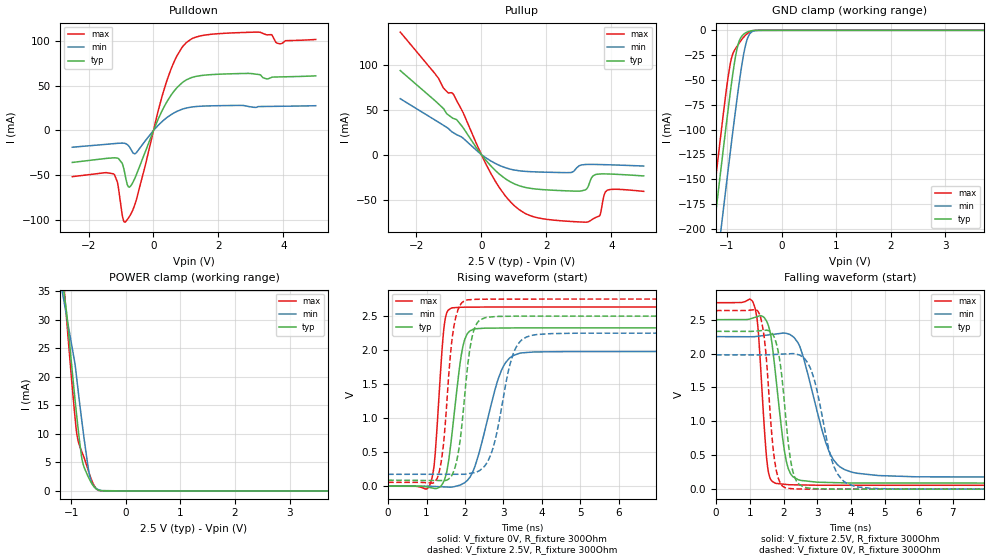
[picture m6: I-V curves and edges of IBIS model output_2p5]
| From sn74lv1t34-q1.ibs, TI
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[Model]   output_2p5
Model_type   Output
Polarity   Non-Inverting
Vmeas = 0.9
Vref = 0.9
Cref = 15pF
Rref = 100000
|   typ   min   max
C_comp   4.947pF   4.835pF   5.043pF
[Voltage Range]   2.5   2.25   2.75
[Temperature Range]   27   125   -40
[Pullup Reference]   2.5   2.25   2.75
[Pulldown Reference]   -0   0   0
[Power Clamp Reference]   2.5   2.25   2.75
[GND Clamp Reference]   0   0   0
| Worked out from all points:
|   slope of the pulldown table from 0 to 0.375 V, typ, clamps not added: 12.6 ohm
|   slope of the pullup table from 0 to 0.375 V, typ, clamps not added: 24 ohm
|   GND clamp passes 1 mA (typ) near -0.59 V on its own axis
|   POWER clamp passes 1 mA (typ) near -0.60 V on its own axis
|   falling waveform, V_fixture 2.5V, R_fixture 300Ohm: 20-80 % time 335ps typ, 676ps min, 207ps max; typ from 2.5 V to 0.088 V
|   rising waveform, V_fixture 0V, R_fixture 300Ohm: 20-80 % time 290ps typ, 552ps min, 186ps max; typ from 0 V to 2.33 V
|   rising waveform, V_fixture 2.5V, R_fixture 300Ohm: 20-80 % time 280ps typ, 452ps min, 240ps max; typ from 0.088 V to 2.5 V
|   falling waveform, V_fixture 0V, R_fixture 300Ohm: 20-80 % time 298ps typ, 523ps min, 252ps max; typ from 2.33 V to 0 V
[Pulldown]
|   Voltage   I(typ)   I(min)   I(max)
-2.5V     -35.79mA   -18.74mA   -51.7mA
-1.23V    -30.63mA   -14.75mA   -48.54mA
-1.114V   -30.88mA   -14.41mA   -57.55mA
-956.5mV  -37.5mA    -14.14mA   -95.94mA
-872.5mV  -50.05mA   -14.51mA   -102.7mA
-683.5mV  -61.25mA   -21.9mA    -92.7mA
-536.5mV  -50.33mA   -25.2mA    -78.68mA
387.5mV   30.58mA    13.77mA    53.11mA
1.018V    56.81mA    25.22mA    98.68mA
3.159V    63.05mA    25.84mA    110.2mA
3.905V    60.03mA    27.12mA    97.04mA
5.28V     NA         NA         NA
[GND Clamp]
|   Voltage   I(typ)   I(min)   I(max)
-2.5V     -817.8mA   -872.3mA   -789.1mA
-1.303V   -231.2mA   -292.1mA   -196.1mA
-1.23V    -196.2mA   -257.3mA   -160.8mA
-1.125V   -146.7mA   -208.1mA   -111.2mA
-1.062V   -117.5mA   -178.9mA   -82.22mA
-946mV    -65.86mA   -126.2mA   -35.86mA
-830.5mV  -22.76mA   -75.49mA   -17.36mA
-767.5mV  -9.785mA   -49.8mA    -12.22mA
-694mV    -3.965mA   -24.23mA   -6.893mA
-589mV    -891.1uA   -3.999mA   -1.764mA
-431.5mV  -12.85uA   -82.5uA    -10.97uA
8V        0A         0A         0A
[Pullup]
|   Voltage   I(typ)   I(min)   I(max)
-2.5V     93.52mA    62.21mA    136.3mA
-1.177V   51.48mA    32.8mA     74.46mA
-872.5mV  40.36mA    24.61mA    67.72mA
429.5mV   -17.63mA   -9.806mA   -29.65mA
1.312V    -36.14mA   -18.49mA   -64.67mA
2.75V     -40.43mA   -19.9mA    -74.3mA
3.275V    -36.4mA    -10.9mA    -74.93mA
3.433V    -23.71mA   -10.89mA   -71.59mA
3.643V    -21.51mA   -11.02mA   -68.06mA
3.779V    -21.44mA   -11.14mA   -45.04mA
3.873V    -21.49mA   -11.24mA   -39.63mA
5.28V     NA         NA         NA
[POWER Clamp]
|   Voltage   I(typ)   I(min)   I(max)
-2.5V     142.8mA    115.5mA    175.3mA
-1.167V   37.39mA    35.21mA    40.36mA
-1.083V   31.33mA    30.63mA    30.15mA
-935.5mV  16.74mA    22.66mA    13.62mA
-904mV    13.8mA     20.34mA    10.62mA
-883mV    11.92mA    18.58mA    9.292mA
-799mV    5.487mA    11.92mA    6.762mA
-757mV    4.04mA     8.831mA    5.712mA
-662.5mV  2.013mA    2.787mA    2.926mA
-589mV    837.6uA    921.3uA    1.128mA
-494.5mV  114.2uA    194.6uA    87.23uA
8V        0A         0A         0A
[Ramp]
R_load = 300
|   typ   min   max
dV/dt_r   1.39637/2.89983e-10   1.18808/5.507e-10   1.58042/1.85495e-10
dV/dt_f   1.44698/3.33617e-10   1.24493/6.73372e-10   1.61611/2.0617e-10
[Falling Waveform]
V_fixture = 2.5V
V_fixture_min = 2.25V
V_fixture_max = 2.75V
R_fixture = 300Ohm
C_fixture = 0F
|   Time   V(typ)   V(min)   V(max)
0s        2.5V       2.25V      2.75V
1.136ns   2.531V     2.249V     2.703V
1.249ns   2.549V     2.256V     2.348V
1.522ns   2.452V     2.273V     353.9mV
1.741ns   1.797V     2.287V     91.27mV
2.018ns   588.3mV    2.302V     72.43mV
2.221ns   216.9mV    2.27V      64.78mV
3.34ns    98.56mV    564.5mV    57.79mV
4.014ns   91.09mV    251.9mV    57.71mV
15ns      88.36mV    175.1mV    56.48mV
[Rising Waveform]
V_fixture = 0V
V_fixture_min = 0V
V_fixture_max = 0V
R_fixture = 300Ohm
C_fixture = 0F
|   Time   V(typ)   V(min)   V(max)
0s        3.396uV    3.144uV    3.15uV
1.101ns   -20.53mV   -1.038mV   39.04mV
1.22ns    -33.89mV   -3.902mV   434.5mV
1.451ns   73.9mV     -9.484mV   2.309V
1.638ns   651.2mV    -13.49mV   2.616V
1.875ns   1.814V     16.57mV    2.63V
2.052ns   2.233V     80.31mV    2.631V
2.947ns   2.324V     1.699V     2.633V
3.415ns   2.326V     1.953V     2.633V
15ns      2.327V     1.98V      2.634V
[Rising Waveform]
V_fixture = 2.5V
V_fixture_min = 2.25V
V_fixture_max = 2.75V
R_fixture = 300Ohm
C_fixture = 0F
|   Time   V(typ)   V(min)   V(max)
0s        88.36mV    175.1mV    56.48mV
1.276ns   83.48mV    175.3mV    113.8mV
1.434ns   82.88mV    175.4mV    581.9mV
1.697ns   205.1mV    175.4mV    2.292V
2.014ns   1.459V     177.7mV    2.731V
2.347ns   2.421V     220.4mV    2.747V
2.726ns   2.49V      553mV      2.749V
3.249ns   2.498V     1.934V     2.75V
3.735ns   2.5V       2.216V     2.75V
15ns      2.5V       2.25V      2.75V
[Falling Waveform]
|Gnd
V_fixture = 0V
V_fixture_min = 0V
V_fixture_max = 0V
R_fixture = 300Ohm
C_fixture = 0F
|   Time   V(typ)   V(min)   V(max)
0s        2.327V     1.98V      2.634V
1.286ns   2.336V     1.98V      2.584V
1.467ns   2.344V     1.98V      2.058V
1.741ns   2.219V     1.987V     404.8mV
2.048ns   1.149V     1.994V     21.5mV
2.428ns   88.13mV    1.984V     3.239mV
2.902ns   8.09mV     1.628V     404.1uV
3.534ns   601.5uV    284.6mV    383.2uV
4.074ns   573.4uV    46.92mV    365.3uV
15ns      3.396uV    3.144uV    3.15uV
